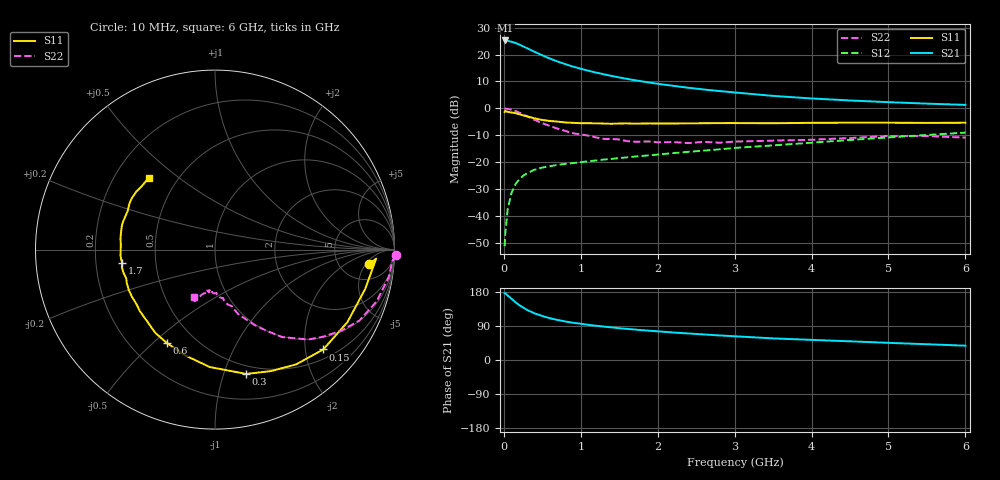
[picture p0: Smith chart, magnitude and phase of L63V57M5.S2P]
!  INFINEON TECHNOLOGIES Small Signal Semiconductors
! BFR380L3 , Si-NPN RF-Transistor in TSLP-3-1
!  Vce=3.5 V,  Ic=7.5 mA
! Common Emitter S-Parameters:  07. March 2005
#  GHz  S  MA  R  50
! f  S11  S21  S12  S22
! GHz  Mag  Ang  Mag  Ang  Mag  Ang  Mag  Ang
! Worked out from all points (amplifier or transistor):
!   36 points, 10 MHz to 6 GHz, reference 50 ohm
!   highest |S21| = 25.2 dB at 20 MHz (marker M1)
!   |S21| within 3 dB of that: start of sweep to 309.7 MHz
!   unconditionally stable (mu >= 1): 2.347 GHz to 4.69 GHz
!   at 250 MHz: K = 0.21, MSG = 24.0 dB, |S12| = -25.0 dB
!   at 1.4 GHz: K = 0.82, MSG = 15.4 dB, |S12| = -18.7 dB
!   at 6 GHz: K = 0.95, MSG = 5.1 dB, |S12| = -9.0 dB
!   S11 on the Smith chart (normalised r, x): 10 MHz: 10, -6; 150 MHz: 0.70, -2.38; 300 MHz: 0.42, -1.19; 600 MHz: 0.35, -0.56; 1.7 GHz: 0.32, -0.07; 6 GHz: 0.35, +0.39
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0.01  0.8605 -5.4  18.16 176.2  0.0028 81.0  1.009 -1.8
0.02  0.8991 -3.2  18.23 176.3  0.005 93.3  0.989 -3.8
0.05  0.865 -14.7  17.89 170.3  0.0136 84.6  0.9807 -9.1
0.1  0.8413 -28.7  17.2 161.4  0.0272 77.5  0.9455 -17.8
0.15  0.8206 -42.7  16.39 152.6  0.0391 68.9  0.8971 -26.1
0.2  0.7831 -54.8  15.3 144.9  0.0488 64.6  0.8389 -32.4
0.25  0.7452 -65.3  14.2 138.5  0.0562 59.2  0.7745 -38.8
0.3  0.7142 -75.9  13.1 132.4  0.0632 55.9  0.7213 -44.0
0.4  0.6549 -92.6  11.22 123.0  0.0733 50.6  0.6144 -52.5
0.5  0.6121 -105.9  9.658 116.0  0.0802 48.0  0.5337 -57.7
0.6  0.5858 -117.1  8.385 110.1  0.0851 46.0  0.4726 -62.5
0.7  0.5708 -125.7  7.414 105.6  0.09 45.4  0.4223 -66.3
0.8  0.5494 -133.8  6.63 101.6  0.0938 44.9  0.3828 -70.1
1.1  0.5322 -150.5  5 92.7  0.1053 46.2  0.3134 -77.0
1.4  0.52 -162.2  4.004 86.1  0.1162 47.8  0.2724 -82.0
1.7  0.5225 -171.7  3.343 80.5  0.1282 50.2  0.2421 -88.0
2.2  0.5255 177.1  2.629 72.6  0.1486 53.4  0.2382 -93.4
2.8  0.5354 166.1  2.104 64.9  0.1746 56.8  0.2318 -101.0
3.5  0.5321 156.1  1.71 57.0  0.2067 58.1  0.2537 -104.8
4.5  0.545 148.2  1.406 49.3  0.2606 60.3  0.2831 -108.8
5.5  0.5398 138.7  1.229 41.6  0.3224 59.4  0.3074 -112.4
6  0.5444 132.8  1.164 37.8  0.3567 58.1  0.2884 -114.2
